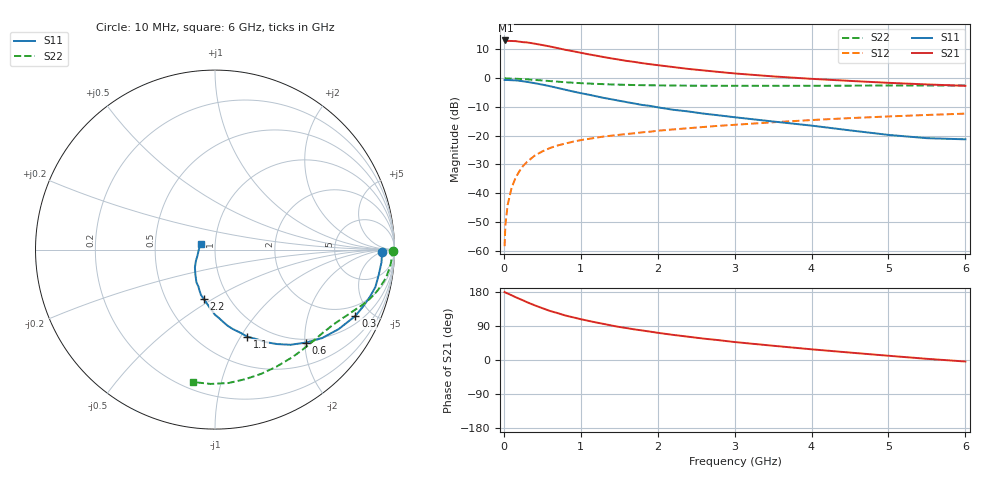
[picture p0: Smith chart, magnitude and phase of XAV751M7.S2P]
! SIEMENS Discrete & RF Semiconductors
! BFY180
! Si NPN RF Bipolar Junction Transistor in MICRO-X
! VCE = 0.75 V  IC = 1.7 mA
! Common Emitter S-Parameters:  May  1997
# GHz  S  MA  R  50
!  f  S11  S21  S12  S22
! GHz  MAG  ANG  MAG  ANG  MAG  ANG  MAG  ANG
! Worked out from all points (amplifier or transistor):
!   36 points, 10 MHz to 6 GHz, reference 50 ohm
!   highest |S21| = 13.1 dB at 20 MHz (marker M1)
!   |S21| within 3 dB of that: start of sweep to 756.6 MHz
!   unconditionally stable (mu >= 1): 1.534 GHz to end of sweep
!   at 250 MHz: K = 0.20, MSG = 21.5 dB, |S12| = -30.5 dB
!   at 1.4 GHz: K = 0.95, MSG = 13.4 dB, |S12| = -20.0 dB
!   at 6 GHz: K = 1.28, MAG = 1.7 dB, |S12| = -12.3 dB
!   S11 on the Smith chart (normalised r, x): 10 MHz: 28, -5; 300 MHz: 1.37, -4.01; 600 MHz: 0.93, -2.03; 1.1 GHz: 0.81, -1.07; 2.2 GHz: 0.76, -0.46; 6 GHz: 0.85, +0.06
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0.01  0.9321 -0.7  4.436 179.4  0.0012 93.8  0.9894 -0.3
0.02  0.9304 -1.7  4.533 178.0  0.0028 86.0  0.9989 -0.8
0.05  0.9304 -4.3  4.456 175.5  0.0063 84.3  0.9877 -1.9
0.1  0.9232 -8.6  4.438 170.9  0.0123 85.4  0.9835 -3.9
0.15  0.9177 -13.1  4.412 166.1  0.0182 81.9  0.9804 -5.7
0.3  0.8648 -25.3  4.193 152.6  0.0349 73.9  0.9552 -10.9
0.4  0.8194 -32.7  3.988 144.4  0.045 69.1  0.935 -14.0
0.5  0.7738 -39.6  3.774 136.8  0.0533 64.8  0.9135 -16.7
0.6  0.7258 -45.5  3.56 129.4  0.0611 61.6  0.8917 -19.1
0.8  0.6297 -56.7  3.115 117.4  0.0731 56.0  0.8507 -23.1
1  0.549 -65.2  2.77 107.7  0.0838 51.7  0.8201 -26.7
1.1  0.5181 -69.6  2.605 103.3  0.0879 50.2  0.8079 -28.1
1.3  0.4541 -77.3  2.329 95.1  0.0968 47.6  0.7881 -31.1
1.5  0.4052 -83.6  2.102 87.2  0.1036 45.5  0.7724 -34.1
1.7  0.3625 -90.1  1.918 80.7  0.1104 44.0  0.7599 -36.9
2.2  0.2826 -102.6  1.564 66.3  0.1285 40.1  0.7461 -44.2
2.6  0.2419 -111.1  1.363 56.4  0.1419 37.6  0.7402 -49.8
3  0.2095 -119.6  1.21 47.4  0.1548 34.6  0.7372 -55.4
3.5  0.1767 -128.2  1.075 37.6  0.1713 31.3  0.7368 -62.4
4.5  0.1238 -149.3  0.898 19.6  0.2024 23.0  0.7414 -76.8
5.5  0.0906 -179.0  0.779 3.1  0.2295 14.5  0.7488 -91.8
6  0.0865 158.2  0.737 -4.0  0.242 9.8  0.7478 -99.3
